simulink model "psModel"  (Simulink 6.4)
settings: Solver=ode45  StartTime=psSimStruct.psSimPar.tStart  StopTime=psSimStruct.psSimPar.tStop  MaxStep=psSimStruct.psSimPar.maxStep  RelTol=psSimStruct.psSimPar.relTol
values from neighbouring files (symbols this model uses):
  psSimStruct = []    [psStartUp.m]
undefined symbols (not defined in the file or in its folder): psVolume

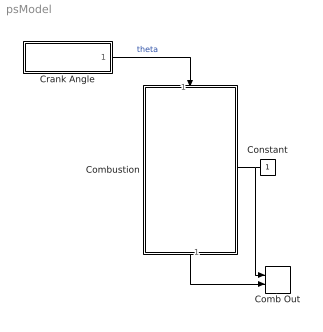
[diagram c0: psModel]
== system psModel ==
  Comb Out : M-S-Function  FunctionName=psToWorkspace  Parameters=6+2*psSimStruct.psThermProp.K,int16('pcb Vb Tb Vu Tu'),1
  Combustion : Subsystem  Orientation=down  TreatAsAtomicUnit=on
  Constant : Constant  Orientation=left
  Crank Angle : Subsystem
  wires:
  Crank Angle/1(theta [rad]) -> Combustion/1(theta)  "theta"
  Combustion/1(IntOut) -> Comb Out/2
  Constant/1 -> Combustion/Enable, Comb Out/1

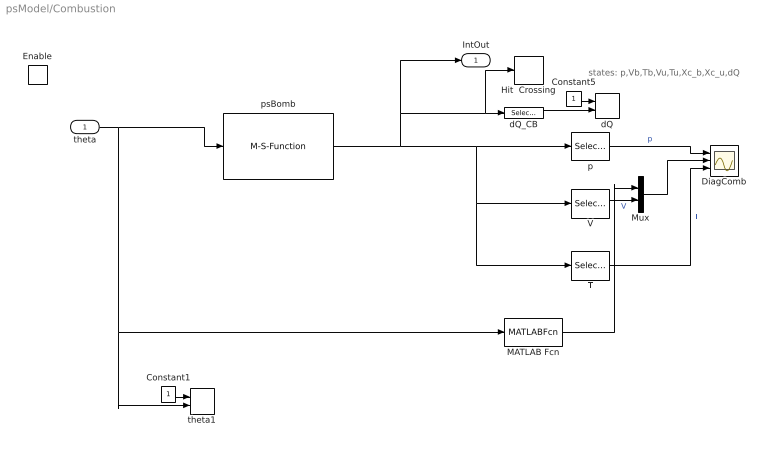
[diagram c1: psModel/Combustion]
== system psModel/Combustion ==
  note: states: p,Vb,Tb,Vu,Tu,Xc_b,Xc_u,dQ
  theta : Inport
  Enable : EnablePort  Orientation=left  StatesWhenEnabling=reset
  Constant1 : Constant
  Constant5 : Constant
  DiagComb : Scope  NumInputPorts=3
  Hit  Crossing : HitCross  HitCrossingDirection=falling
  MATLAB Fcn : MATLABFcn  MATLABFcn=psVolume(u(1))  OutputDimensions=1
  Mux : Mux  Inputs=2
  T : Selector  Elements=[3 5]  Rows=[3 5]  OutputPortSize=[(-2)]
  V : Selector  Elements=[2 4]  Rows=[2 4]  OutputPortSize=[(-2)]
  dQ : M-S-Function  FunctionName=psToWorkspace  Parameters=1,int16('dQ'),1
  dQ_CB : Selector  Elements=[psSimStruct.psThermProp.K*2+6]  Rows=[psSimStruct.psThermProp.K*2+9]  OutputPortSize=[(-2)]
  p : Selector  Elements=[1]  Rows=[1]  OutputPortSize=[(-2)]
  psBomb : M-S-Function  FunctionName=psBomb
  theta1 : M-S-Function  FunctionName=psToWorkspace  Parameters=1,int16('theta'),1
  IntOut : Outport
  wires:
  dQ_CB/1 -> dQ/2
  Constant5/1 -> dQ/1
  psBomb/1 -> IntOut/1, dQ_CB/1, Hit  Crossing/1, p/1, V/1, T/1
  p/1 -> DiagComb/1  "p"
  T/1 -> DiagComb/3  "T"
  V/1 -> Mux/2  "V"
  Mux/1 -> DiagComb/2
  MATLAB Fcn/1 -> Mux/1
  theta/1 -> psBomb/1, MATLAB Fcn/1, theta1/2
  Constant1/1 -> theta1/1

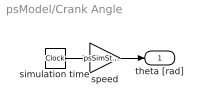
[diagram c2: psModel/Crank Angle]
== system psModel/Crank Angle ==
  simulation time : Clock
  speed : Gain  Gain=psSimStruct.psSimPar.w
  theta [rad] : Outport
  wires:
  speed/1 -> theta [rad]/1
  simulation time/1 -> speed/1
